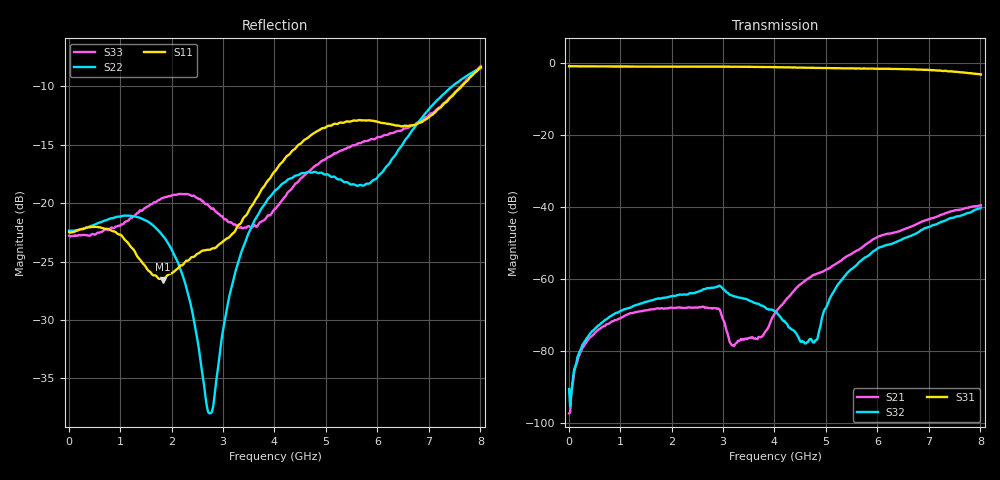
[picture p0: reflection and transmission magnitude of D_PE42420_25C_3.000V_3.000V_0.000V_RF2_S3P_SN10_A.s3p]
! Device ID: PE42420
! Serial: 10
! Insertion: A
! Temp: 25C
! VDD: 3.000
! Control_Hi: 3.000
! Control_Lo: 0.000
! Logic State: RF2
! Port 1: RFC
! Port 2: RF1
! Port 3: RF2
! V1 = 0.00
! V2 = 3.00
! V3 = 0.00
! IDD: 1.126883e-04
#  Hz  S  RI  R  50
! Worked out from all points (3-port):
!   401 points, 10 MHz to 8.01 GHz, reference 50 ohm
!   strongest paths, dB at 10 MHz, 2.01 GHz, 4.01 GHz, 6.01 GHz, 8.01 GHz:
!     S31: -0.8, -0.9, -1.1, -1.5, -3.1
!     S32: -90.7, -64.8, -69.0, -51.4, -40.2
!     S21: -97.4, -68.0, -69.6, -48.2, -39.5
!   lowest |S11| = -26.5 dB at 1.83 GHz (marker M1), VSWR 1.10, Z = 54.5 - j2.02 ohm
!   |S11| at or under -10 dB: start of sweep to 7.635 GHz
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1e7  0.0751 -0.00173  -6.52e-07 -6.06e-06  0.9091 -0.00581
     1.27e-05 -4.48e-06  0.0763 -0.00101  -2.59e-05 -4.78e-06
     0.9108 -0.0047  -1.96e-05 -2.17e-05  0.0725 -0.00135
1.83e9  0.0433 -0.0185  0.000205 0.000334  0.7201 -0.5359
        0.000202 0.000331  0.0633 -0.0356  0.000342 0.000427
        0.718 -0.5375  0.000335 0.00043  0.101 -0.0296
2.75e9  0.053 -0.0344  0.000284 0.000273  0.5117 -0.7367
        0.000283 0.000272  -0.00282 -0.0123  0.000617 0.000423
        0.5085 -0.7384  0.000613 0.000428  0.0704 -0.0654
3.19e9  0.0236 -0.0704  7.88e-05 9.22e-05  0.3886 -0.8074
        8.01e-05 8.86e-05  -0.0454 -0.00643  0.000557 0.000145
        0.3865 -0.8077  0.000563 0.000153  0.0236 -0.078
4.01e9  -0.1004 -0.0935  -0.000298 0.000142  0.1415 -0.8708
        -0.0003 0.000144  -0.1129 -0.00855  0.000324 9.39e-05
        0.1429 -0.8723  0.000344 8.75e-05  -0.0572 -0.0751
4.51e9  -0.1762 -0.0369  -0.000743 0.000387  -0.00371 -0.8719
        -0.000747 0.000395  -0.1336 -0.00756  5.22e-05 0.000128
        -0.00524 -0.8698  7.35e-05 0.000111  -0.1047 -0.0731
4.79e9  -0.2008 0.013  -0.000939 0.000643  -0.0828 -0.8595
        -0.000946 0.000653  -0.1361 -0.00419  -0.000107 0.000138
        -0.0845 -0.8574  -8.06e-05 0.000113  -0.128 -0.0663
5.13e9  -0.2024 0.0784  -0.00126 0.000816  -0.1791 -0.8353
        -0.00127 0.000838  -0.1293 0.0104  -0.000625 0.00025
        -0.1802 -0.8365  -0.000594 0.000212  -0.1545 -0.0461
5.71e9  -0.1537 0.1662  -0.00225 0.00157  -0.3434 -0.7706
        -0.00227 0.0016  -0.1036 0.0584  -0.0015 0.00122
        -0.34 -0.7733  -0.00148 0.00115  -0.1826 0.0121
8.01e9  -0.0813 0.3742  -0.000986 0.0104  -0.6861 -0.1416
        -0.000771 0.0105  0.0201 0.3783  -0.00015 0.00995
        -0.6837 -0.1476  -0.000397 0.0098  -0.0725 0.3794
